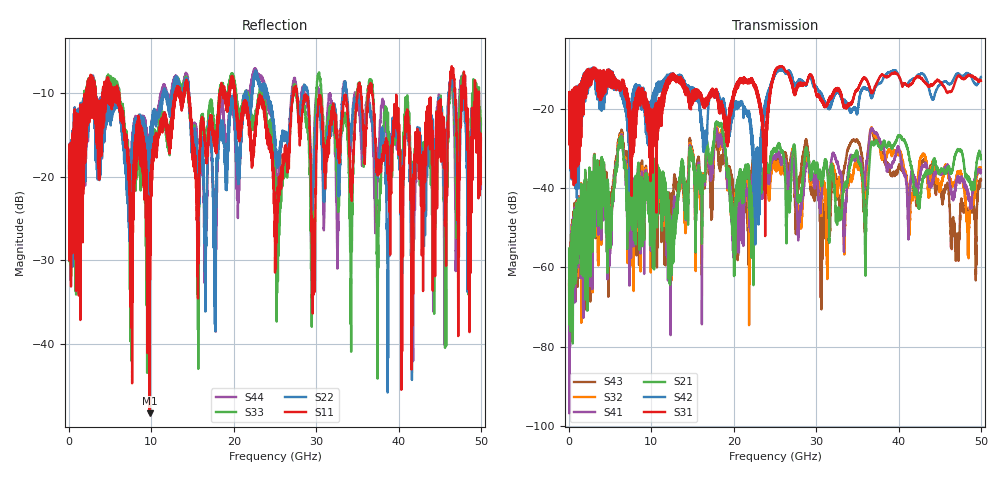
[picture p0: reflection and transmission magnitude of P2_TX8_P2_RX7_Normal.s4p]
!Keysight Technologies,N5225B,MY57041031,A.13.20.10
!Date: Friday, May 31, 2019 11:38:16
!Correction: S11(Full 4 Port(1,2,3,4))
!S12(Full 4 Port(1,2,3,4))
!S13(Full 4 Port(1,2,3,4))
!S14(Full 4 Port(1,2,3,4))
!S21(Full 4 Port(1,2,3,4))
!S22(Full 4 Port(1,2,3,4))
!S23(Full 4 Port(1,2,3,4))
!S24(Full 4 Port(1,2,3,4))
!S31(Full 4 Port(1,2,3,4))
!S32(Full 4 Port(1,2,3,4))
!S33(Full 4 Port(1,2,3,4))
!S34(Full 4 Port(1,2,3,4))
!S41(Full 4 Port(1,2,3,4))
!S42(Full 4 Port(1,2,3,4))
!S43(Full 4 Port(1,2,3,4))
!S44(Full 4 Port(1,2,3,4))
!S4P File: Measurements: <S11,S12,S13,S14>,
!<S21,S22,S23,S24>,
!<S31,S32,S33,S34>,
!<S41,S42,S43,S44>:
# Hz S  dB  R 50.0
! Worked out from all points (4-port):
!   5000 points, 10 MHz to 50 GHz, reference 50 ohm
!   strongest paths, dB at 10 MHz, 12.51 GHz, 25.01 GHz, 37.51 GHz, 50 GHz:
!     S31: -19.4, -11.7, -10.3, -12.8, -12.8
!     S42: -19.3, -12.1, -11.4, -13.7, -11.9
!     S21: -55.2, -56.4, -30.7, -29.1, -32.7
!     S41: -63.4, -50.9, -31.6, -26.8, -35.8
!     S32: -64.3, -53.3, -34.6, -28.1, -35.1
!     S43: -63.4, -43.6, -32.2, -28.0, -37.9
!   lowest |S11| = -48.3 dB at 9.79 GHz (marker M1), VSWR 1.01, Z = 50 - j0.381 ohm
!   |S11| at or under -10 dB: 20.17 GHz to 27.18 GHz (7.011 GHz wide, 29.6 % of centre); 27.67 GHz to 35.04 GHz (7.367 GHz wide, 23.5 % of centre); 36.79 GHz to 46.16 GHz (9.368 GHz wide, 22.6 % of centre)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
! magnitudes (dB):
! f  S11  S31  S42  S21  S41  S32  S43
! 10 MHz  -19.6  -19.4  -19.3  -55.2  -63.4  -64.3  -63.4
! 6.23 GHz  -12.0  -13.7  -14.1  -28.7  -28.3  -27.8  -26.9
! 9.79 GHz  -48.3  -26.2  -18.3  -48.6  -42.8  -43.6  -39.9
! 22.8 GHz  -11.9  -16.0  -36.9  -37.1  -33.6  -33.7  -31.6
! 25.47 GHz  -21.2  -9.4  -10.1  -28.6  -31.5  -33.2  -32.8
! 30.71 GHz  -11.6  -18.3  -16.4  -37.7  -40.8  -43.1  -49.9
! 50 GHz  -15.4  -12.8  -11.9  -32.7  -35.8  -35.1  -37.9
